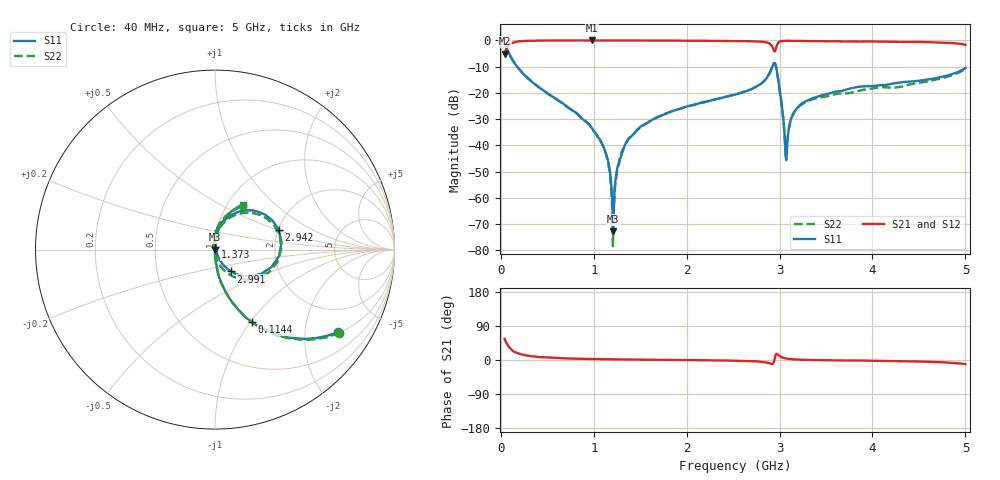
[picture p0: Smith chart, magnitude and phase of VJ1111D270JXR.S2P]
! VJ1111D270JXR
! DATE 02/16/2022  10:20
! CAPACITORS MOUNTED IN SERIES ON 25 MIL THICK MICROSTRIP SUBSTRATE
# GHz  S  MA  R  50.00
!  FREQ  S11M  S11A  S21M  S21A  S12M  S12A  S22M  S22A
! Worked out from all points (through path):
!   801 points, 40 MHz to 5 GHz, reference 50 ohm
!   highest |S21| = -0.01 dB at 982.4 MHz (marker M1); lowest = -5.0 dB at 40 MHz (marker M2)
!   group delay of S21, straight-line fit = 9.2 ps
!   lowest |S11| = -72.8 dB at 1.206 GHz (marker M3), VSWR 1.00, Z = 50 - j0.0171 ohm
!   |S11| at or under -10 dB: 173.7 MHz to 2.922 GHz (2.748 GHz wide, 178 % of centre); 2.962 GHz to end of sweep
!   |S22| runs from -78.5 to -1.6 dB; largest |S21 - S12| = 0.037
!   S11 on the Smith chart (normalised r, x): 40 MHz: 1.02, -2.96; 114.4 MHz: 1.00, -1.02; 1.373 GHz: 1.00, +0.03; 2.942 GHz: 2.02, +0.51; 2.991 GHz: 1.16, -0.29; 5 GHz: 1.18, +0.65
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0.04  0.8259 -34.0  0.5621 55.9  0.5617 55.9  0.8345 -33.8
0.1144  0.4553 -62.9  0.8868 27.4  0.8945 27.2  0.4601 -62.7
0.3438  0.1571 -81.5  0.9873 9.5  0.9931 9.3  0.1583 -81.0
0.8708  0.03283 -88.1  0.9986 3.1  1.004 3.0  0.03283 -88.6
0.9824  0.02096 -89.5  0.999 2.6  1.005 2.4  0.02071 -90.6
1.1312  0.006982 -87.3  0.9977 2.0  1.003 1.8  0.006701 -92.2
1.2056  0.0002293 -48.1  0.9969 1.8  1.002 1.6  0.0001191 2.1
1.2242  0.001584 86.3  0.9977 1.7  1.003 1.5  0.001376 93.0
1.2428  0.002754 85.1  0.9972 1.7  1.002 1.5  0.002467 101.6
1.2738  0.004581 84.0  0.997 1.6  1.003 1.4  0.005212 96.3
1.373  0.01333 87.7  0.9966 1.2  1.002 1.1  0.01316 89.8
1.6954  0.03495 87.7  0.9928 0.5  0.9989 0.3  0.03506 87.3
2.52  0.09254 82.6  0.9751 -1.8  0.9811 -2.0  0.09277 82.4
2.8424  0.1748 71.2  0.9291 -5.9  0.9342 -6.1  0.1748 68.9
2.9416  0.3719 17.0  0.6262 -2.2  0.6301 -2.4  0.3685 12.0
2.9912  0.151 -53.8  0.9227 12.3  0.9281 12.1  0.1485 -62.2
3.0532  0.01677 -58.5  0.9818 4.9  0.9873 4.8  0.01561 -102.7
3.0718  0.005221 29.5  0.9828 4.0  0.9886 3.9  0.005802 162.0
3.1648  0.04496 88.1  0.98 1.6  0.9865 1.4  0.04466 96.8
3.3508  0.07854 86.3  0.9725 -0.1  0.978 -0.2  0.07483 89.0
4.1754  0.1449 77.4  0.947 -2.8  0.9527 -2.9  0.1263 78.8
5  0.2967 57.9  0.8254 -10.8  0.8307 -11.0  0.2865 57.2
